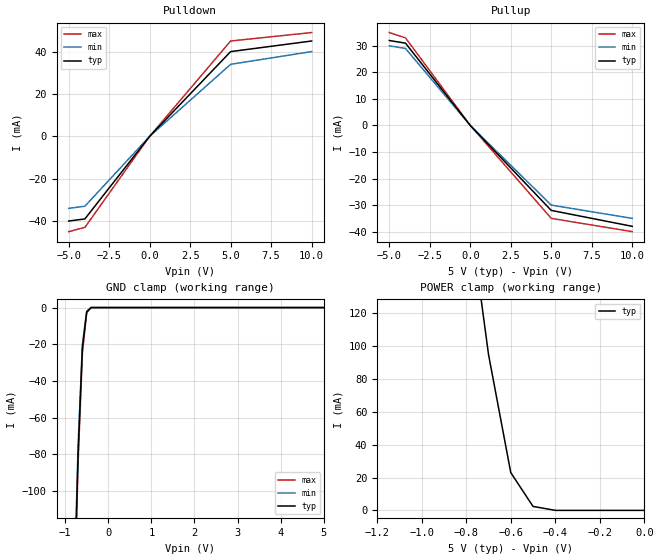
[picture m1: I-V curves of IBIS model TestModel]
|DESCRIPTION OF BUG:
|Use of the the keyword [Add Submodel] instead of [Submodel]
|causes program "hangs."  While text output is generated properly
|identifying the error, the program will not generate a final error
|count and pass/fail verdict.  The program will not end without
|user intervention.
|The enclosed example will "hang" the IBISCHK3 program; however,
|program crashes have been observed with more complex models.
|This bug also applies to DOS32 IBISCHK3 v3.2.5 under Windows 98SE.
[IBIS Ver]   3.2
[File Name]   bug52.ibs
[File Rev]   0.0
[Date]   05-December-2000
[Source]   File created from specification
[Disclaimer]
   (C) Copyright 2000 Intel Corp.
   All rights reserved
   This model is for demonstration purposes only,
[Component]   GENERIC_IBIS
[Manufacturer]   Intel Corp.
[Package]
|   typ   min   max
R_pkg   6.0mO   5.0mO   7.0mO
L_pkg   5.0nH   2.0nH   8.0nH
C_pkg   1.0pF   0.5pF   1.5pF
[Pin]   signal_name   model_name   R_pin   L_pin   C_pin
   1   TestSignal   TestModel
| Models and submodels in the file (1): TestModel (I/O)
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[Model]   TestModel
Model_type   I/O
Polarity   Non-Inverting
Vinl = 800mV
Vinh = 2.0V
Cref = 10.0pF
Vref = 0.0
Rref = 25
Vmeas = 0.4
C_comp   5.00pF   4.00pF   6.00pF
[Temperature Range]   27.00   100.00   0.00
[Voltage Range]   5.0V   4.75V   5.25V
[Add Submodel]
testsub   Non-Driving
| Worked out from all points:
|   slope of the pulldown table from 0 to 0.75 V, typ, clamps not added: 125 ohm
|   slope of the pullup table from 0 to 0.75 V, typ, clamps not added: 156 ohm
|   GND clamp passes 1 mA (typ) near -0.44 V on its own axis
|   POWER clamp passes 1 mA (typ) near -0.44 V on its own axis
[Pulldown]
| voltage   I(typ)   I(min)   I(max)
-5V       -40mA      -34mA      -45mA
-4V       -39mA      -33mA      -43mA
0V        0A         0A         0A
5V        40mA       34mA       45mA
10V       45mA       40mA       49mA
[Pullup]
| voltage   I(typ)   I(min)   I(max)
-5V       32mA       30mA       35mA
-4V       31mA       29mA       33mA
0V        0A         0A         0A
5V        -32mA      -30mA      -35mA
10V       -38mA      -35mA      -40mA
[GND Clamp]
| voltage   I(typ)   I(min)   I(max)
-5V       -3.9A      -3.8A      -4A
-700mV    -80mA      -75mA      -85mA
-600mV    -22mA      -20mA      -25mA
-500mV    -2.4mA     -2mA       -2.9mA
-400mV    0A         0A         0A
5V        0A         0A         0A
[Power Clamp]
| voltage   I(typ)   I(min)   I(max)
-5V       4.45A      NA         NA
-700mV    95mA       NA         NA
-600mV    23mA       NA         NA
-500mV    2.4mA      NA         NA
-400mV    0A         NA         NA
0V        0A         NA         NA
[Ramp]
|variable   typ   min   max
dV/dt_r   2.20/1.06n   1.92/1.28n   2.49/650p
dV/dt_f   2.46/1.21n   2.21/1.54n   2.70/770p
R_load = 300ohms
[Add Submodel]   testsub
Submodel_type  Dynamic_clamp
[GND Clamp]
| voltage   I(typ)   I(min)   I(max)
-5V       -40mA      -34mA      -45mA
-4V       -39mA      -33mA      -43mA
0V        0A         0A         0A
5V        40mA       34mA       45mA
10V       45mA       40mA       49mA
